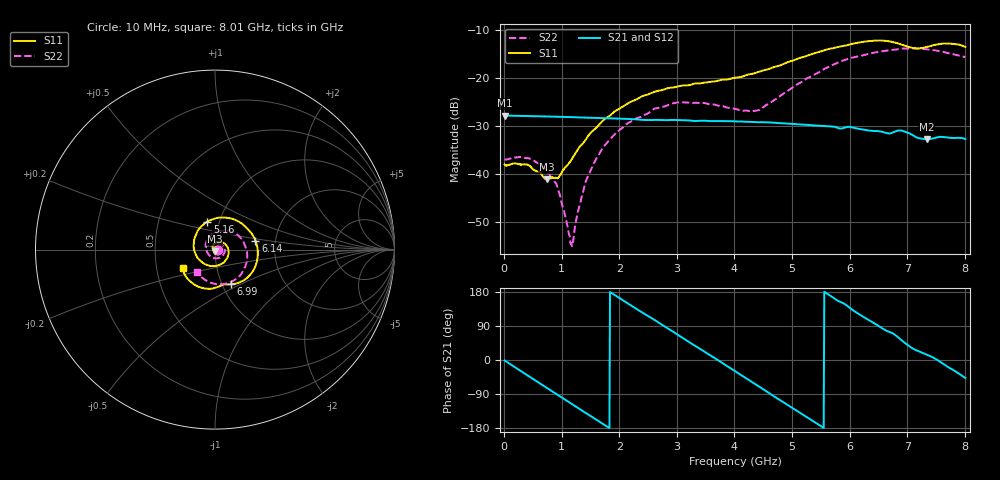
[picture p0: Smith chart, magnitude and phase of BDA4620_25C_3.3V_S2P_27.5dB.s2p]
!Agilent Technologies,E5071B,MY42404982,A.09.10
!Date: Wed May 06 08:54:47 2026
!Data & Calibration Information:
!Freq	S11:SOLT2(ON)	S21:SOLT2(ON)	S12:SOLT2(ON)	S22:SOLT2(ON)
# Hz S RI R 50
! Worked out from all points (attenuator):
!   801 points, 10 MHz to 8.01 GHz, reference 50 ohm
!   highest |S21| = -27.88 dB at 10 MHz (marker M1); lowest = -32.8 dB at 7.34 GHz (marker M2)
!   lowest |S11| = -41.2 dB at 740 MHz (marker M3), VSWR 1.02, Z = 49.9 - j0.87 ohm
!   |S11| at or under -10 dB: start of sweep to end of sweep
!   |S22| runs from -55.1 to -13.9 dB; largest |S21 - S12| = 0.0002
!   S11 on the Smith chart (normalised r, x): 10 MHz: 1.03, -0.00; 5.16 GHz: 0.88, +0.28; 6.14 GHz: 1.57, +0.17; 6.99 GHz: 1.10, -0.44; 8.01 GHz: 0.68, -0.15
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1e7  0.0125 -0.000747  0.0404 -0.000824  0.0404 -0.000844  0.014 -0.000468
4.4e8  0.00902 -0.00814  0.0287 -0.0276  0.0288 -0.0276  0.0135 -0.00509
7.4e8  -0.000759 -0.00872  0.0112 -0.0378  0.0113 -0.0379  0.00801 -0.0072
9.3e8  -0.00728 -0.00522  -0.00134 -0.0391  -0.00138 -0.0392  0.00356 -0.00624
1.17e9  -0.0132 0.00462  -0.0167 -0.035  -0.0167 -0.0351  -0.00153 -0.0011
1.2e9  -0.0136 0.00627  -0.0185 -0.0341  -0.0185 -0.0341  -0.002 -1.2e-05
1.35e9  -0.0141 0.0145  -0.0263 -0.0281  -0.0263 -0.0281  -0.00355 0.00454
1.53e9  -0.0105 0.0255  -0.0333 -0.0188  -0.0333 -0.0188  -0.00341 0.0112
1.77e9  0.00139 0.0377  -0.0376 -0.0041  -0.0377 -0.00408  0.000599 0.0204
2.15e9  0.0329 0.0428  -0.0319 0.019  -0.032 0.019  0.0168 0.0291
2.68e9  0.0728 0.00722  -0.00566 0.0358  -0.00564 0.0359  0.0442 0.0197
3.08e9  0.0697 -0.0439  0.0178 0.0314  0.0179 0.0314  0.0551 -0.00704
4.01e9  -0.0634 -0.077  0.0305 -0.0173  0.0306 -0.0173  -0.0101 -0.0464
4.43e9  -0.1154 -0.00468  0.0116 -0.0323  0.0116 -0.0323  -0.0444 -0.0118
5.16e9  -0.0426 0.1564  -0.0256 -0.0202  -0.0256 -0.0202  -0.0094 0.0887
5.35e9  0.0116 0.1761  -0.03 -0.0109  -0.03 -0.0109  0.023 0.1018
6.14e9  0.2254 0.0502  -0.0161 0.0246  -0.0161 0.0247  0.1626 0.034
6.68e9  0.1835 -0.1537  0.00697 0.0253  0.00702 0.0254  0.17 -0.0897
6.99e9  0.0872 -0.1929  0.0202 0.0179  0.0203 0.0179  0.1262 -0.1566
7.34e9  0.017 -0.2074  0.0221 0.00549  0.0222 0.0056  0.0429 -0.1928
7.66e9  -0.0907 -0.2079  0.0233 -0.00585  0.0233 -0.00582  -0.035 -0.1798
8.01e9  -0.1803 -0.1052  0.0155 -0.0169  0.0156 -0.017  -0.1015 -0.1275
